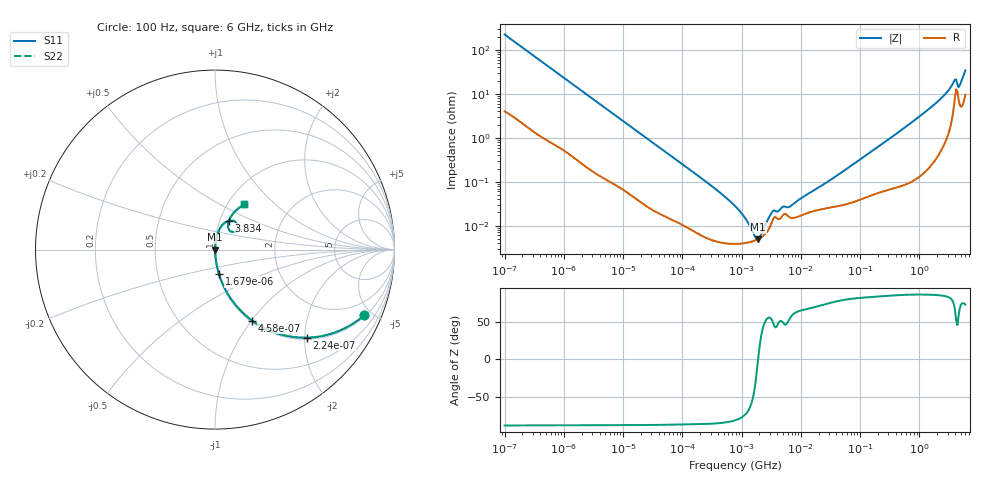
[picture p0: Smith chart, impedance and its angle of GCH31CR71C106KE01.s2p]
!Murata Part Number: GCH31CR71C106KE01
!These Parameters are Measured in Series Mode Connection
!Data Generated on Jun 19, 2026
!  o--ll--o
!Port1  Port2
!  o------o
!Operation Temp=25[degC], DC Bias Voltage=0[V]
!Freq. Start=100[Hz] Stop=6[GHz] 401[Steps]
# Hz S RI R 50
!Freq.(Hz) S11(Real) S11(Imag) S21(Real) S21(Imag) S12(Real) S12(Imag) S22(Real) S22(Imag)
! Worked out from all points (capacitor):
!   401 points, 100 Hz to 6 GHz, reference 50 ohm
!   read as one part in series: C = 7 uF near 109 Hz
!   lowest |Z| = 4.93 mohm at 1.897 MHz (marker M1)
!   series resonance near 1.901 MHz, so ESL is about 1 nH
!   S11 on the Smith chart (normalised r, x): 100 Hz: 1.08, -4.52; 224 Hz: 1.04, -2.04; 458 Hz: 1.02, -1.01; 1.679 kHz: 1.01, -0.28; 3.834 GHz: 1.10, +0.37; 6 GHz: 1.19, +0.66
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100  0.832 -0.3651  0.168 0.3651  0.168 0.3651  0.832 -0.3651
224  0.5104 -0.4907  0.4896 0.4907  0.4896 0.4907  0.5104 -0.4907
458  0.2063 -0.3951  0.7937 0.3951  0.7937 0.3951  0.2063 -0.3951
820  0.0789 -0.2591  0.9211 0.2591  0.9211 0.2591  0.0789 -0.2591
1679  0.0221 -0.1363  0.9779 0.1363  0.9779 0.1363  0.0221 -0.1363
2008  0.016 -0.115  0.984 0.115  0.984 0.115  0.016 -0.115
6433  0.00231 -0.037  0.9977 0.037  0.9977 0.037  0.00231 -0.037
40335  0.000226 -0.0061  0.9998 0.0061  0.9998 0.0061  0.000226 -0.0061
302498  4.83e-05 -0.000825  1 0.000825  1 0.000825  4.83e-05 -0.000825
774597  3.84e-05 -0.000278  1 0.000278  1 0.000278  3.84e-05 -0.000278
1386327  4.22e-05 -8.8e-05  1 8.8e-05  1 8.8e-05  4.22e-05 -8.8e-05
1896632  4.93e-05 -7e-07  1 7e-07  1 7e-07  4.93e-05 -7e-07
2481164  6.37e-05 7.73e-05  0.9999 -7.73e-05  0.9999 -7.73e-05  6.37e-05 7.73e-05
3394479  0.000139 0.000165  0.9999 -0.000165  0.9999 -0.000165  0.000139 0.000165
6644369  0.000152 0.00023  0.9998 -0.00023  0.9998 -0.00023  0.000152 0.00023
1.555665e7  0.00021 0.000567  0.9998 -0.000567  0.9998 -0.000567  0.00021 0.000567
3.124326e8  0.000751 0.00948  0.9992 -0.00948  0.9992 -0.00948  0.000751 0.00948
1.873145e9  0.00676 0.0598  0.9932 -0.0598  0.9932 -0.0598  0.00676 0.0598
3.065283e9  0.0248 0.113  0.9752 -0.113  0.9752 -0.113  0.0248 0.113
3.8344e9  0.0766 0.1613  0.9234 -0.1613  0.9234 -0.1613  0.0766 0.1613
4.796499e9  0.0714 0.1263  0.9286 -0.1263  0.9286 -0.1263  0.0714 0.1263
6e9  0.1637 0.253  0.8363 -0.253  0.8363 -0.253  0.1637 0.253
